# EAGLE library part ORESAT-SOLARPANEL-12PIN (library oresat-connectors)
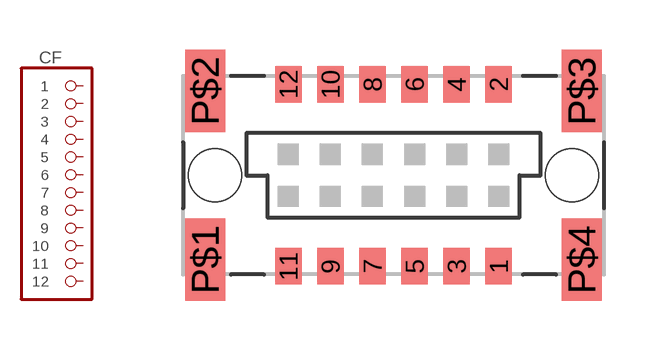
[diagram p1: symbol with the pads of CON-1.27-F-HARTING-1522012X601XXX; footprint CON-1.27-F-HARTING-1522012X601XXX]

Designator prefix CF

## ORESAT-SOLARPANEL-12PIN  [CON-1.27-F-HARTING-1522012X601XXX]
1  1  pas
2  2  pas
3  3  pas
4  4  pas
5  5  pas
6  6  pas
7  7  pas
8  8  pas
9  9  pas
10  10  pas
11  11  pas
12  12  pas

## Footprint CON-1.27-F-HARTING-1522012X601XXX (pad centres in mm)
smd 0.8 x 1.1: 1 3.175,-2.75; 2 3.175,2.75; 3 1.905,-2.75; 4 1.905,2.75; 5 0.635,-2.75; 6 0.635,2.75; 7 -0.635,-2.75; 8 -0.635,2.75; 9 -1.905,-2.75; 10 -1.905,2.75; 11 -3.175,-2.75; 12 -3.175,2.75
smd 1.2 x 2.5: P$1 -5.685,-2.55; P$2 -5.685,2.55; P$3 5.685,2.55; P$4 5.685,-2.55
hole 1.6 at -5.385,0
hole 1.6 at 5.385,0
